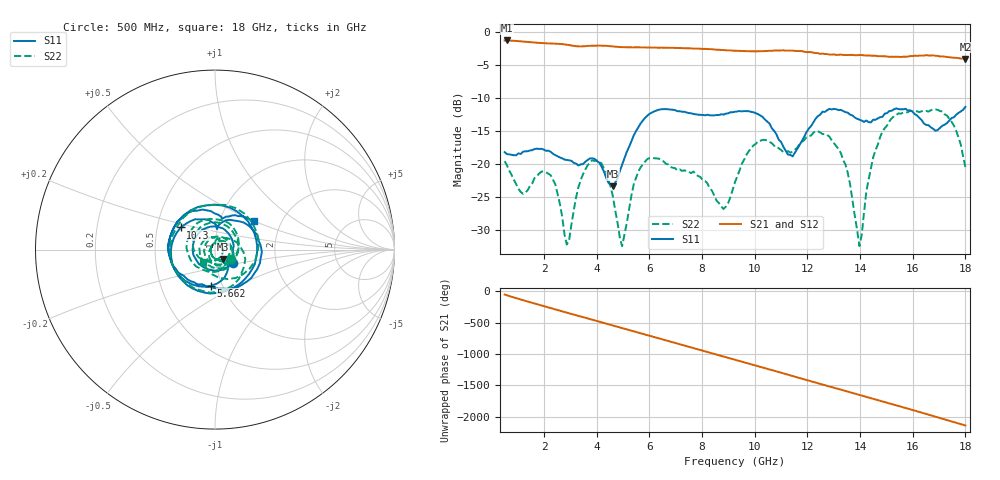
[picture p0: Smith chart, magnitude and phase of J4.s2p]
!Agilent Technologies,N5230A,MY45001360,A.07.50.67
!Agilent N5230A: A.07.50.67
!Date: Tuesday, April 16, 2024 15:54:13
!Correction: S11(Full 2 Port(1,2))
!S21(Full 2 Port(1,2))
!S12(Full 2 Port(1,2))
!S22(Full 2 Port(1,2))
!S2P File: Measurements: S11, S21, S12, S22:
# Hz S  dB  R 50
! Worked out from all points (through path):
!   201 points, 500 MHz to 18 GHz, reference 50 ohm
!   highest |S21| = -1.32 dB at 587.5 MHz (marker M1); lowest = -4.1 dB at 18 GHz (marker M2)
!   group delay of S21, straight-line fit = 330 ps
!   lowest |S11| = -23.4 dB at 4.612 GHz (marker M3), VSWR 1.15, Z = 54.3 - j5.65 ohm
!   |S11| at or under -10 dB: start of sweep to end of sweep
!   |S22| runs from -32.4 to -11.7 dB; largest |S21 - S12| = 0.008
!   S11 on the Smith chart (normalised r, x): 500 MHz: 1.20, -0.18; 5.662 GHz: 0.89, -0.37; 10.3 GHz: 0.66, +0.17; 18 GHz: 1.45, +0.51
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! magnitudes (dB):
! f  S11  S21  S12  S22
! 500 MHz  -18.2  -1.3  -1.3  -19.6
! 587.5 MHz  -18.5  -1.3  -1.3  -20.2
! 1.2 GHz  -18.1  -1.5  -1.5  -24.5
! 2.25 GHz  -18.1  -1.8  -1.8  -21.7
! 2.862 GHz  -19.4  -2.0  -1.9  -32.1
! 3.475 GHz  -20.0  -2.2  -2.2  -21.6
! 4.088 GHz  -19.7  -2.1  -2.1  -19.5
! 4.612 GHz  -23.4  -2.2  -2.2  -24.9
! 4.963 GHz  -20.1  -2.3  -2.3  -32.4
! 5.662 GHz  -13.9  -2.4  -2.3  -20.5
! 6.362 GHz  -11.8  -2.4  -2.4  -19.2
! 8.812 GHz  -12.5  -2.8  -2.8  -26.8
! 9.25 GHz  -12.1  -2.9  -2.9  -22.7
! 10.3 GHz  -12.9  -2.9  -2.9  -16.3
! 11.44 GHz  -18.8  -2.9  -2.9  -18.1
! 12.22 GHz  -13.7  -3.2  -3.1  -15.3
! 13.45 GHz  -12.2  -3.5  -3.5  -20.1
! 13.97 GHz  -13.3  -3.5  -3.5  -32.4
! 14.5 GHz  -13.3  -3.6  -3.6  -18.9
! 15.11 GHz  -12.0  -3.8  -3.7  -13.5
! 17.12 GHz  -14.2  -3.7  -3.8  -12.0
! 18 GHz  -11.3  -4.1  -4.1  -20.4
